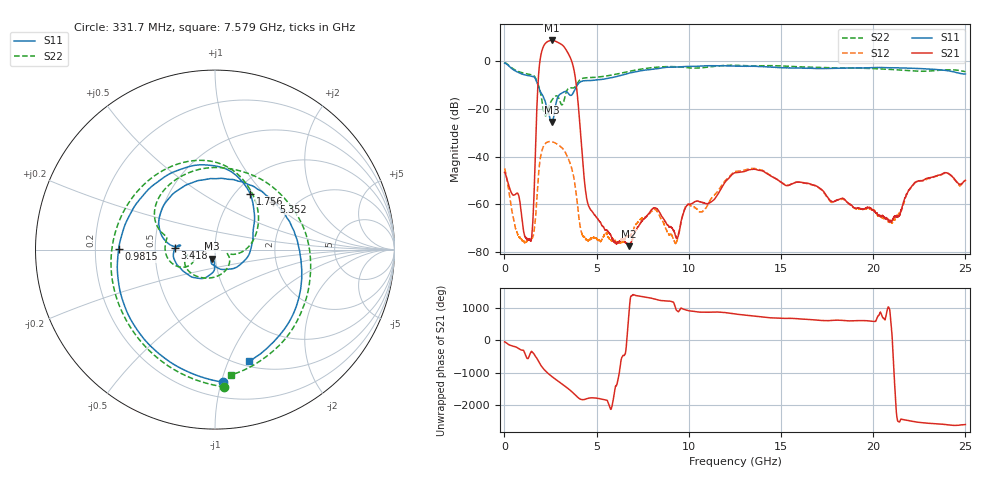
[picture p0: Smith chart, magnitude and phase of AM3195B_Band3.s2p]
!Agilent Technologies,E8364B,MY43040894,A.07.50.67
!Agilent E8364B: A.07.50.67
!Date: Wednesday, July 07, 2021 13:17:23
!Correction: S11(Full 2 Port(1,2))
!S21(Full 2 Port(1,2))
!S12(Full 2 Port(1,2))
!S22(Full 2 Port(1,2))
!S2P File: Measurements: S11, S21, S12, S22:
# Hz S  dB  R 50
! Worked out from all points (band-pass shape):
!   8001 points, 10 MHz to 25 GHz, reference 50 ohm
!   highest |S21| = 8.75 dB at 2.565 GHz (marker M1); lowest = -77.5 dB at 6.751 GHz (marker M2)
!   |S21| within 3 dB of the highest: 2.09 GHz to 3.267 GHz (1.177 GHz wide, 44 % of centre)
!   lowest |S11| = -25.4 dB at 2.565 GHz (marker M3), VSWR 1.11, Z = 48.2 - j4.93 ohm
!   |S11| at or under -10 dB: 1.813 GHz to 3.947 GHz (2.133 GHz wide, 74.1 % of centre)
!   |S22| runs from -22.8 to -0.5 dB; largest |S21 - S12| = 2.8
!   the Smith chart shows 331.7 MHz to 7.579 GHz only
!   S11 on the Smith chart (normalised r, x): 331.7 MHz: 0.31, -1.01; 981.5 MHz: 0.30, +0.00; 1.756 GHz: 1.16, +0.84; 3.418 GHz: 0.63, +0.01; 5.352 GHz: 1.56, +1.02; 7.579 GHz: 0.55, -1.19
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1e7  -0.75 -13.2  -46.54 -40.9  -44.85 -38.8  -0.50 -14.1
3.317462e8  -2.62 -86.5  -54.27 -153.7  -59.09 -154.1  -2.31 -86.1
9.814862e8  -5.40 179.7  -67.91 60.2  -75.10 -55.0  -4.81 179.8
1.45942e9  -6.19 118.5  -74.79 16.8  -74.34 40.1  -5.59 120.2
1.756176e9  -8.68 57.9  -20.08 171.3  -58.04 -17.4  -8.20 60.2
2.05918e9  -14.13 -2.6  5.09 -113.6  -36.82 76.6  -17.60 -9.4
2.33407e9  -20.04 -84.0  8.26 79.1  -33.84 -87.9  -21.19 -26.6
2.565228e9  -25.42 -107.6  8.75 -31.3  -33.70 163.4  -16.34 -89.8
2.721415e9  -20.90 -91.3  8.56 -99.2  -34.09 96.2  -14.87 -124.9
2.902592e9  -14.91 -116.3  7.94 -174.1  -34.90 22.5  -14.84 -158.8
3.130626e9  -13.28 -149.9  6.89 92.5  -36.29 -68.6  -18.21 -160.0
3.418011e9  -13.02 178.2  3.88 -31.4  -39.97 171.8  -11.81 -164.3
3.677282e9  -13.86 175.3  -0.62 -155.2  -45.62 49.8  -11.19 168.8
4.177082e9  -8.41 137.0  -35.07 -26.3  -71.57 101.5  -7.32 134.9
5.351612e9  -7.51 39.4  -69.29 -22.6  -73.69 46.3  -6.36 37.3
6.751052e9  -4.97 -39.4  -77.47 123.3  -73.27 -54.4  -4.22 -44.8
7.578846e9  -3.74 -73.3  -65.93 -91.7  -65.47 -107.4  -3.05 -82.9
8.341041e9  -3.04 -101.3  -62.34 172.2  -63.68 166.2  -2.44 -113.2
1.2505e10  -1.99 141.2  -46.70 100.7  -46.23 101.4  -1.67 127.0
1.667208e10  -2.94 19.8  -51.69 -77.1  -51.73 -79.3  -2.50 3.9
2.083604e10  -2.70 -69.0  -66.76 -47.1  -67.33 -103.8  -3.34 -81.0
2.5e10  -5.32 -124.2  -49.84 -80.1  -50.17 -79.0  -4.34 -132.9
